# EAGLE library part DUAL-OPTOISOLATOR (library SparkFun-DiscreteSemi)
Optocoupler, Phototransistor Output, Dual Channel Optically coupled pairs with a gallium arsenide infrared LED and a silicon NPN phototransistor. Signal information, including a DC level, can be transmitted by the device while maintaining a high degree of electrical isolation between input and output.
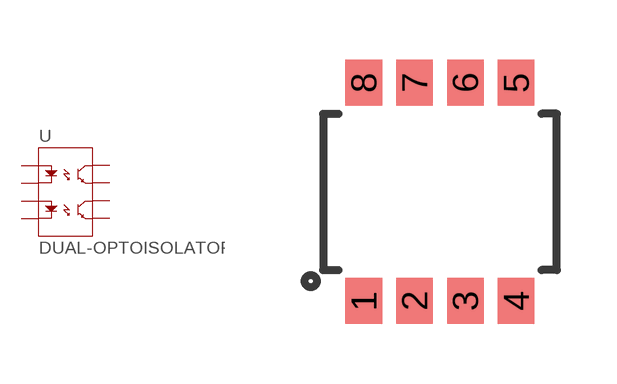
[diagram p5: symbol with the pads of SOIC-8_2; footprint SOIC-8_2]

Designator prefix U

## DUAL-OPTOISOLATORSOIC8 (PROD_ID: IC-09076)  [SOIC-8_2]
1  A1
2  C1
3  A2
4  C2
5  EM2
6  CL2
7  EM1
8  CL1

## Footprint SOIC-8_2 (pad centres in mm)
smd 0.914 x 1.143: 1 -1.905,-2.731; 2 -0.635,-2.731; 3 0.635,-2.731; 4 1.905,-2.731; 5 1.905,2.731; 6 0.635,2.731; 7 -0.635,2.731; 8 -1.905,2.731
